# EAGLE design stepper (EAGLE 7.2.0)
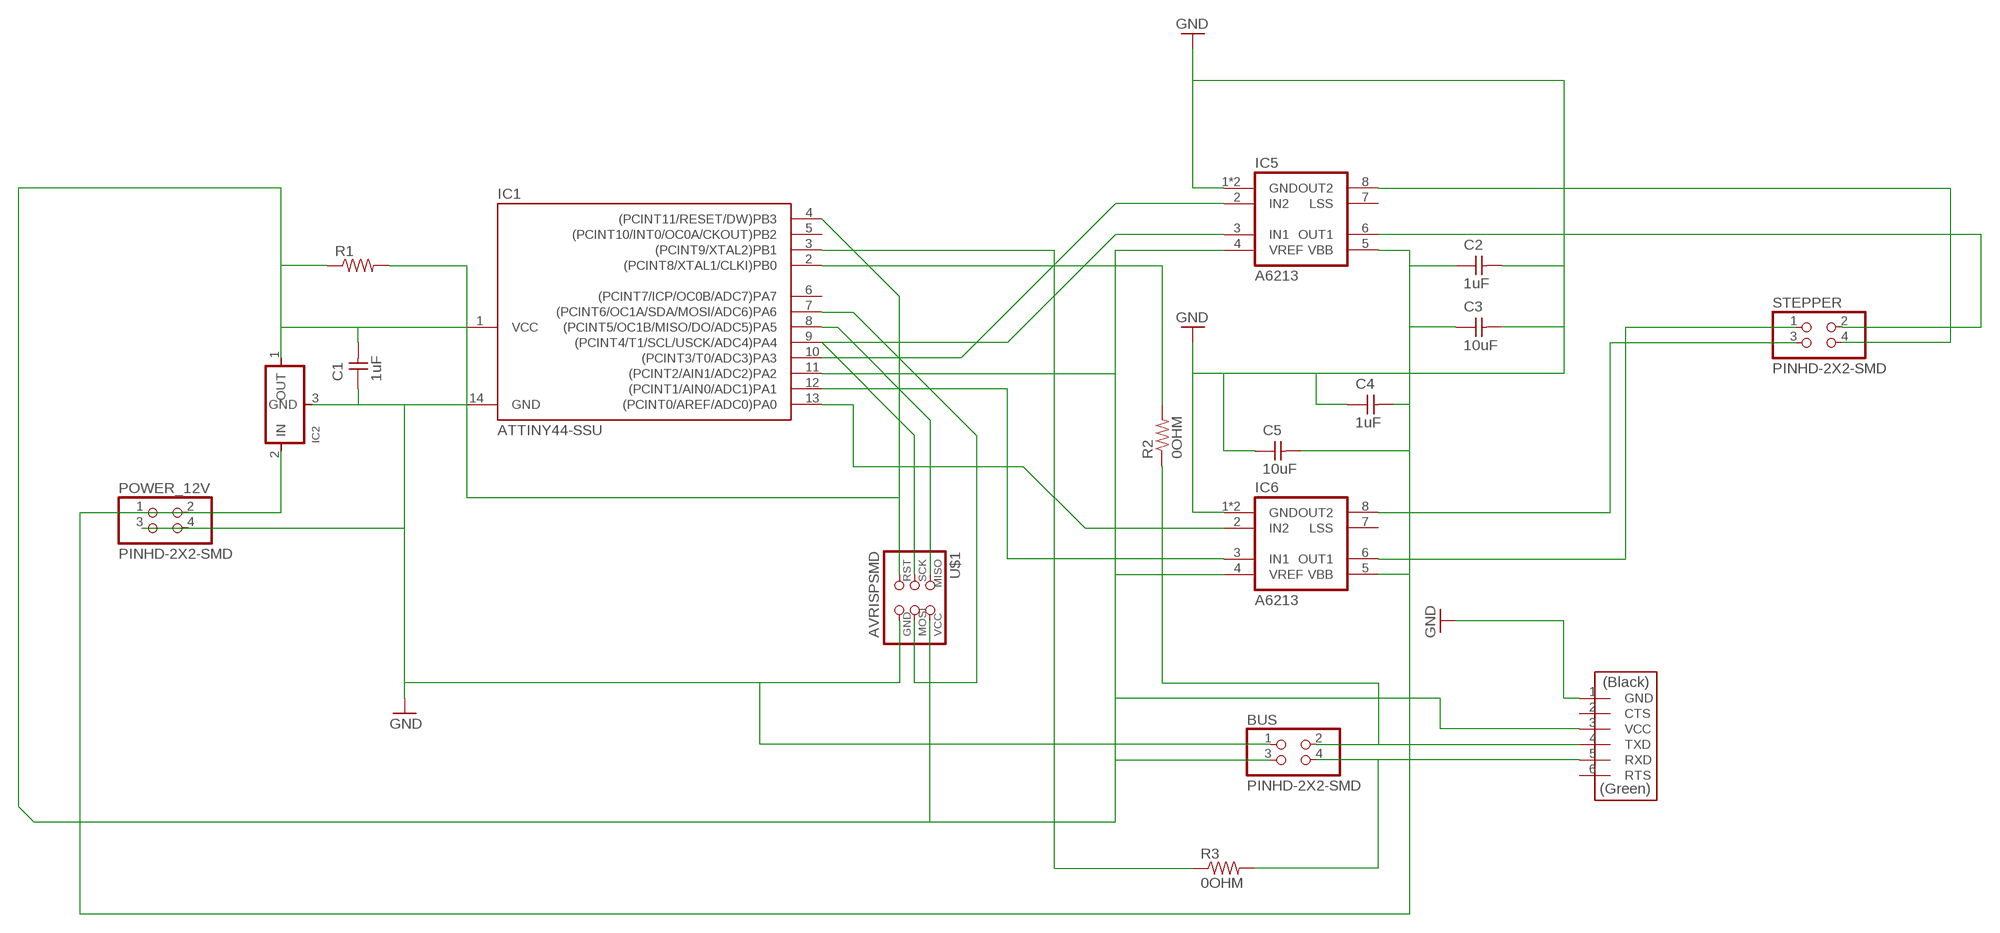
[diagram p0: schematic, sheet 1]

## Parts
BUS  PINHD-2X2-SMD  [2X02SMD]
C1  1uF  CAP-UNPOLARIZEDFAB  [C1206FAB]
C2  1uF  CAP-UNPOLARIZEDFAB  [C1206FAB]
C3  10uF  CAP-UNPOLARIZEDFAB  [C1206FAB]
C4  1uF  CAP-UNPOLARIZEDFAB  [C1206FAB]
C5  10uF  CAP-UNPOLARIZEDFAB  [C1206FAB]
IC1  ATTINY44-SSU  [SOIC14]
IC2  REGULATORSOT23  [SOT23]
IC5  A6213  [SOIC08]
IC6  A6213  [SOIC08]
POWER_12V  PINHD-2X2-SMD  [2X02SMD]
R1  RES-US1206FAB  [R1206FAB]
R2  0OHM  RES-US1206FAB  [R1206FAB]
R3  0OHM  RES-US1206FAB  [R1206FAB]
STEPPER  PINHD-2X2-SMD  [2X02SMD]
U$1  AVRISPSMD  [2X03SMD]
U$2  FTDI-SMD-HEADER  [1X06SMD]

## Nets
0OUM: BUS.2 R2.1 U$2.4(TXD)
GND: BUS.1 C1.1 C2.2 C3.2 C4.1 C5.1 IC1.14(GND) IC2.3(GND) IC5.1(GND) IC5.TP(GND) IC6.1(GND) IC6.TP(GND) POWER_12V.3 POWER_12V.4 U$1.6(GND) U$2.1(GND)
N$1: C2.1 C3.1 C4.2 C5.2 IC2.2(IN) IC5.5(VBB) IC6.5(VBB) POWER_12V.1 POWER_12V.2
N$2: BUS.3 C1.2 IC1.1(VCC) IC1.11((PCINT2/AIN1/ADC2)PA2) IC2.1(OUT) IC5.4(VREF) IC6.4(VREF) R1.1 U$1.2(VCC) U$2.3(VCC)
N$3: IC1.4((PCINT11/RESET/DW)PB3) R1.2 U$1.5(RST)
N$4: IC1.9((PCINT4/T1/SCL/USCK/ADC4)PA4) IC5.3(IN1) U$1.3(SCK)
N$5: IC1.8((PCINT5/OC1B/MISO/DO/ADC5)PA5) U$1.1(MISO)
N$6: IC1.7((PCINT6/OC1A/SDA/MOSI/ADC6)PA6) U$1.4(MOSI)
N$7: IC1.13((PCINT0/AREF/ADC0)PA0) IC6.2(IN2)
N$8: IC1.12((PCINT1/AIN0/ADC1)PA1) IC6.3(IN1)
N$9: IC1.10((PCINT3/T0/ADC3)PA3) IC5.2(IN2)
N$10: IC1.2((PCINT8/XTAL1/CLKI)PB0) R2.2
N$11: IC1.3((PCINT9/XTAL2)PB1) R3.1
N$12: IC6.8(OUT2) STEPPER.3
N$13: IC6.6(OUT1) STEPPER.1
N$14: IC5.8(OUT2) STEPPER.4
N$15: IC5.6(OUT1) STEPPER.2
N$17: BUS.4 R3.2 U$2.5(RXD)
Unconnected: IC1.5((PCINT10/INT0/OC0A/CKOUT)PB2) IC1.6((PCINT7/ICP/OC0B/ADC7)PA7) IC5.7(LSS) IC6.7(LSS) U$2.2(CTS) U$2.6(RTS)

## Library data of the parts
BUS POWER_12V STEPPER = 01_fab:PINHD-2X2-SMD
C1-C5 = 01_fab:CAP-UNPOLARIZED
IC1 = 01_fab:ATTINY44
IC2 = 01_fab:REGULATOR
IC5 IC6 = 01_allegro-a4953:A6213: The A6213 is a single IC switching regulator that provides constant-current output to drive high-power LEDs. It integrates a high-side N-channel DMOS switch for DC-to-DC step- down (buck) conversion. A true average current is output using a cycle-by-cycle, controlled on-time method. The library has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
R1-R3 = 01_fab:RES-US: Resistor (US Symbol)
U$1 = 01_fab:AVRISP
U$2 = 01_fab:FTDI-SMD-HEADER

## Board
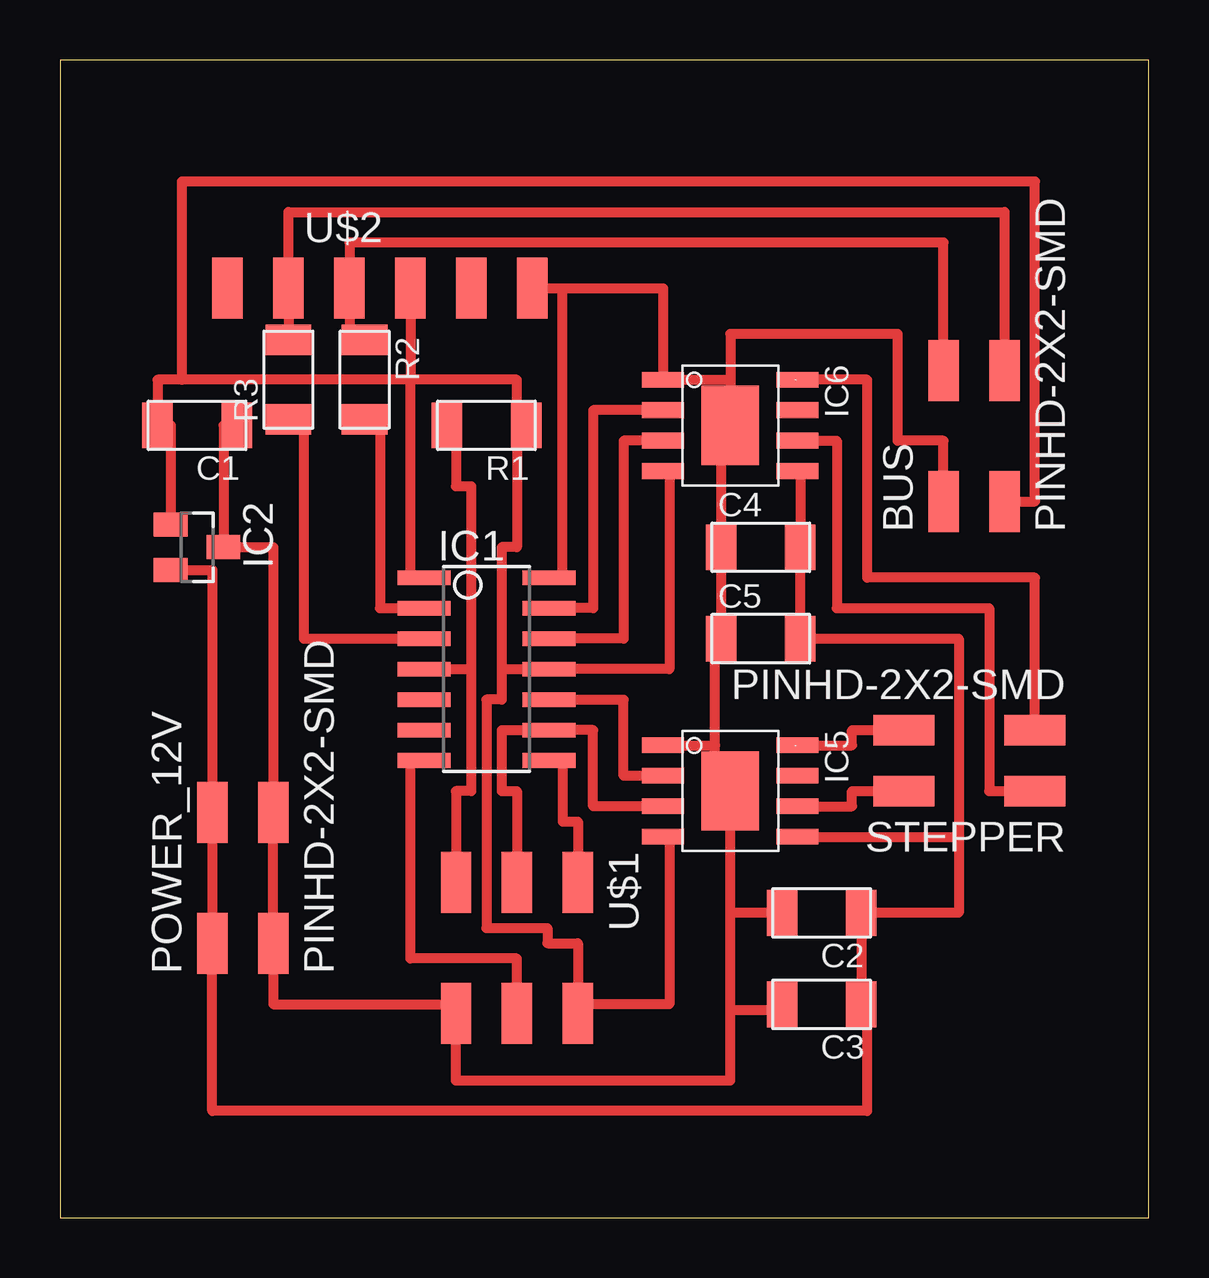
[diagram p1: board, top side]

Size 45.39 x 48.25 mm. Coordinates in mm from the lower left corner, seen from the top.
Outline: 0,0 45.39,0 45.39,48.25 0,48.25 0,0
Copper layers (1*16): Top 0.035mm / dielectric 1.5mm / Bottom 0.035mm
Design rules "default": minimum track width 10mil, minimum drill 24mil, track to track 8mil, track to pad 8mil, pad to pad 8mil, via to via 8mil, smd to smd 8mil, copper to edge 40mil, drill to drill 8mil, minimum pad ring 10mil, minimum via ring 8mil, stop-mask expansion 4mil, vias tented up to drill 0mil, thermal gap 10mil

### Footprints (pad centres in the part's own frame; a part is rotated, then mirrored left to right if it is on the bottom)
2X02SMD = smd 2.54 x 1.27: 1 -2.54,1.27; 2 2.92,1.27; 3 -2.54,-1.27; 4 2.92,-1.27
C1206FAB = smd 1.27 x 1.905: 1 -1.651,0; 2 1.651,0
SOIC14 = smd 0.61 x 2.21: 1 -3.81,-2.603; 2 -2.54,-2.603; 3 -1.27,-2.603; 4 0,-2.603; 5 1.27,-2.603; 6 2.54,-2.603; 7 3.81,-2.603; 8 3.81,2.603; 9 2.54,2.603; 10 1.27,2.603; 11 0,2.603; 12 -1.27,2.603; 13 -2.54,2.603; 14 -3.81,2.603
SOT23 = smd 1 x 1.4: 1 -0.95,-1.1; 2 0.95,-1.1; 3 0,1.1
SOIC08 = smd 0.65 x 1.75: 1 -1.905,-2.8; 2 -0.635,-2.8; 3 0.635,-2.8; 4 1.905,-2.8; 5 1.905,2.8; 6 0.635,2.8; 7 -0.635,2.8; 8 -1.905,2.8 | smd 3.3 x 2.41: TP 0,0
R1206FAB = smd 1.27 x 1.905: 1 -1.651,0; 2 1.651,0
2X03SMD = smd 2.54 x 1.27: 1 -2.54,2.54; 2 2.92,2.54; 3 -2.54,0; 4 2.92,0; 5 -2.54,-2.54; 6 2.92,-2.54
1X06SMD = smd 2.54 x 1.27: 1 0,6.35; 2 0,3.81; 3 0,1.27; 4 0,-1.27; 5 0,-3.81; 6 0,-6.35

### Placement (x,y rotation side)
BUS  38.1,32.39 90 top
C1  5.71,33.02 180 top
C2  31.75,12.7 180 top
C3  31.75,8.89 180 top
C4  29.21,27.94 0 top
C5  29.21,24.13 0 top
IC1  17.78,22.86 270 top
IC2  5.71,27.94 270 top
IC5  27.94,17.78 270 top
IC6  27.94,33.02 270 top
POWER_12V  7.62,13.97 90 top
R1  17.78,33.02 180 top
R2  12.7,34.92 270 top
R3  9.52,34.92 90 top
STEPPER  38.1,19.05 180 top
U$1  19.05,11.43 270 top
U$2  13.34,38.73 270 top

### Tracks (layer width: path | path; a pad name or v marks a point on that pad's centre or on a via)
0OUM
  Top 0.406: BUS.2 36.83,40.64 12.07,40.64 U$2.4 12.07,36.19 12.7,36.19 R2.1
GND
  Top 0.406: C3.2 29.85,8.64 27.94,8.64 | 27.31,19.69 27.31,17.78 IC5.TP 27.94,12.7 | 27.31,19.69 27.31,23.88 C5.1 C4.1 27.56,33.02 IC6.TP 27.94,34.92 | IC5.1 27.31,19.69 | C1.1 6.82,33.02 IC2.3 8.89,27.94 POWER_12V.4 POWER_12V.3 8.89,8.89 16.51,8.89 U$1.6 16.51,5.72 27.94,5.72 27.94,8.64 | U$2.1 20.95,38.73 | 20.95,38.73 25.14,38.73 IC6.1 27.94,34.92 | IC1.14 20.95,26.67 20.95,38.73 | BUS.1 36.83,32.39 34.92,32.39 34.92,36.83 27.94,36.83 27.94,34.92 | 27.94,12.7 27.94,8.89 27.94,8.64 | C2.2 27.94,12.7
N$1
  Top 0.406: 37.47,15.88 37.47,12.7 C2.1 C3.1 33.66,8.89 33.66,4.45 6.35,4.45 POWER_12V.1 POWER_12V.2 6.35,26.99 IC2.2 | IC6.5 30.86,31.12 C4.2 C5.2 37.47,24.13 37.47,15.88 | IC5.5 37.47,15.88
N$2
  Top 0.406: IC2.1 4.62,33.02 C1.2 4.06,34.92 5.08,34.92 | 19.05,33.02 19.05,34.92 14.61,34.92 | 14.61,34.92 5.08,34.92 | R1.1 19.05,33.02 | 19.05,33.02 19.05,27.94 18.41,27.94 18.41,22.86 | 18.41,22.86 IC1.11 25.4,22.86 25.4,31.12 IC6.4 | IC1.1 14.61,26.67 14.61,34.92 | IC5.4 25.4,15.88 25.4,8.89 21.59,8.89 U$1.2 21.59,11.43 20.32,11.43 20.32,12.06 17.78,12.06 17.78,21.59 18.41,21.59 18.41,22.86 | U$2.3 14.61,34.92 | BUS.3 40.64,29.84 40.64,43.18 5.08,43.18 5.08,34.92
N$3
  Top 0.406: R1.2 16.51,32.64 16.51,30.48 17.14,30.48 17.14,22.86 | IC1.4 17.14,22.86 | 17.14,22.86 17.14,17.78 16.51,17.78 U$1.5
N$4
  Top 0.406: IC5.3 22.22,17.15 22.22,20.32 IC1.9 18.41,20.32 18.41,17.78 19.05,17.78 U$1.3
N$5
  Top 0.406: 20.32,19.05 IC1.8 20.95,19.05 20.95,16.51 21.59,16.51 U$1.1
N$6
  Top 0.406: U$1.4 19.05,10.8 14.61,10.8 14.61,19.05 IC1.7
N$7
  Top 0.406: IC1.13 22.22,25.4 22.22,33.66 IC6.2
N$8
  Top 0.406: IC1.12 23.5,24.13 23.5,31.75 23.5,32.39 IC6.3
N$9
  Top 0.406: IC1.10 23.5,21.59 23.5,18.41 IC5.2
N$10
  Top 0.406: R2.2 13.34,33.27 13.34,25.4 IC1.2
N$11
  Top 0.406: R3.1 10.16,33.27 10.16,24.13 IC1.3
N$12
  Top 0.406: STEPPER.3 40.64,26.67 33.66,26.67 33.66,34.92 IC6.8
N$13
  Top 0.406: IC6.6 32.39,32.39 32.39,25.4 38.73,25.4 38.73,17.78 STEPPER.1
N$14
  Top 0.406: IC5.8 33.02,19.69 33.02,20.32 STEPPER.4
N$15
  Top 0.406: IC5.6 33.02,17.15 33.02,17.78 STEPPER.2
N$17
  Top 0.406: R3.2 U$2.5 9.52,41.91 39.37,41.91 BUS.4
